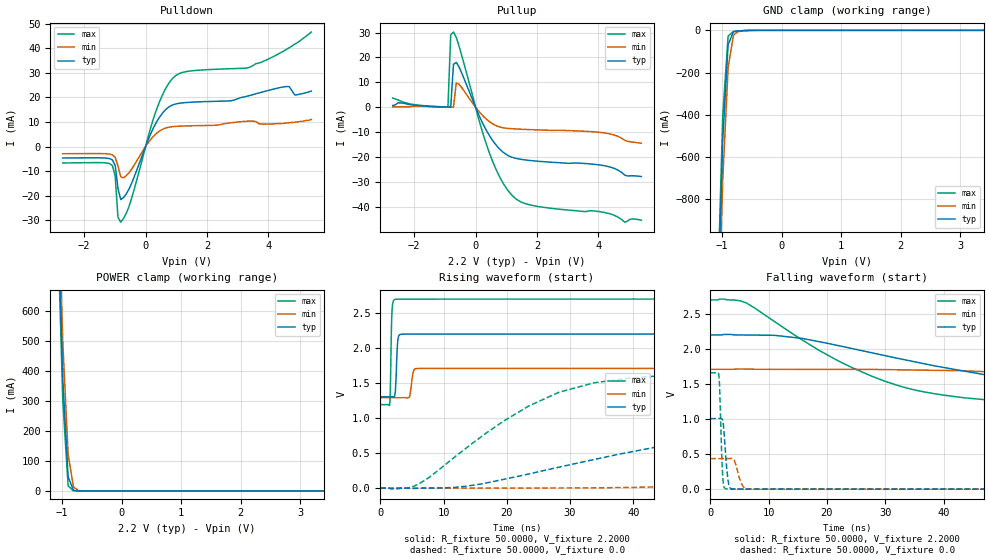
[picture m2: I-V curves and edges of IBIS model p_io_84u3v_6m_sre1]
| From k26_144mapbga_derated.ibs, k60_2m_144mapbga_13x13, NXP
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[Model] p_io_84u3v_6m_sre1
|   Model p_io_84u3v_6m_sre1
| Library cells for typ/min/max conditions are connected as defined below:
|  pad - External Pad
|  ipp_do - Core Input
|  ipp_obe - Output Buffer Enable
|  esd_boost - vdd_s_3v
|  esd_bus - vdd_s_3v
|  ipp_ina40a_3v - NC
|  ipp_ina40b_3v - NC
|  ipp_ina_3v - NC
|  ipp_ind - NC
|  ipp_ind_3v - NC
|  ipp_sre - vdd_s_lv
|  vdd_s_3v - vdd_s_3v
|  vdd_s_lv - vdd_s_lv
|  vss_bulk - vss_bulk
|  vss_s_lv - vss_s_lv
| All other pins connected to ground
Model_type I/O
Polarity   Non-Inverting
Enable   Active-High
Vinl =   0.6600V
Vinh =   1.6500V
Vmeas =  1.1000V
Cref =   25.0000pF
Rref =   50.0000
Vref =   0.0V
C_comp   2.2801pF   2.0930pF   2.5126pF
[Temperature Range]   25.0000   0.1250k   -40.0000
[Voltage Range]   2.2000V   1.7100V   2.7000V
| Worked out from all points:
|   slope of the pulldown table from 0 to 0.33 V, typ, clamps not added: 35.3 ohm
|   slope of the pullup table from 0 to 0.33 V, typ, clamps not added: 37.5 ohm
|   GND clamp passes 1 mA (typ) near -0.60 V on its own axis
|   POWER clamp passes 1 mA (typ) near -0.77 V on its own axis
|   rising waveform, R_fixture 50.0000, V_fixture 2.2000: 20-80 % time 249ps typ, 365ps min, 188ps max; typ from 1.3 V to 2.2 V
|   rising waveform, R_fixture 50.0000, V_fixture 0.0: 20-80 % time 37.7ns typ, 81.3ns min, 17ns max; typ from 0 V to 1.01 V
|   falling waveform, R_fixture 50.0000, V_fixture 2.2000: 20-80 % time 36.7ns typ, 76.7ns min, 20.7ns max; typ from 2.2 V to 1.3 V
|   falling waveform, R_fixture 50.0000, V_fixture 0.0: 20-80 % time 571ps typ, 930ps min, 381ps max; typ from 1.01 V to 0 V
[Pulldown]
|Voltage   I(typ)   I(min)   I(max)
-2.7V     -4.67mA    -2.93mA    -6.69mA
-1.08V    -5.482mA   -3.411mA   -7.784mA
-990mV    -7.73mA    -4.407mA   -11.96mA
-900mV    -17mA      -7.855mA   -28.73mA
-810mV    -21.6mA    -12.32mA   -30.8mA
-540mV    -17.32mA   -10.67mA   -24.41mA
360mV     10.04mA    5.403mA    15.15mA
900mV     17.03mA    8.127mA    28.01mA
3.33V     20.57mA    10.32mA    32.05mA
4.59V     24.4mA     9.6mA      39.55mA
4.86V     21mA       9.9mA      41.7mA
5.4V      22.6mA     11mA       46.6mA
[Pullup]
|Voltage   I(typ)   I(min)   I(max)
-2.7V     700uA      200uA      3.7mA
-900mV    67.5uA     41uA       85.4uA
-810mV    41.47uA    24.4uA     29.06mA
-720mV    17.26mA    23.27uA    30.18mA
-630mV    17.97mA    9.767mA    28.09mA
450mV     -11.38mA   -5.776mA   -18.35mA
810mV     -17.11mA   -8.025mA   -28.58mA
1.17V     -20.02mA   -8.615mA   -35.14mA
1.89V     -21.53mA   -9.048mA   -39.53mA
4.05V     -23.2mA    -10.08mA   -41.95mA
4.86V     -27.27mA   -13.28mA   -46.17mA
5.4V      -27.86mA   -14.46mA   -45.4mA
[GND_clamp]
|Voltage   I(typ)   I(min)   I(max)
-2.7V     -22.06A    -21.95A    -22.16A
-1.08V    -1.367A    -1.534A    -1.279A
-990mV    -516.1mA   -705.4mA   -403.6mA
-900mV    -68.3mA    -177.8mA   -27.24mA
-810mV    -6.453mA   -22.51mA   -5.196mA
-720mV    -2.652mA   -3.714mA   -3.053mA
-450mV    -86.98uA   -164.9uA   -52.14uA
5.4V      0A         0A         0A
[POWER_clamp]
|Voltage   I(typ)   I(min)   I(max)
-2.7V     15.08A     14.99A     15.18A
-1.08V    969.6mA    1.072A     917.9mA
-990mV    374.4mA    496mA      302.2mA
-900mV    47.23mA    122mA      16.99mA
-810mV    1.773mA    12.96mA    214.5uA
-720mV    53.91uA    987.1uA    2.438uA
-630mV    1.624uA    71.95uA    27.87nA
5.4V      0A         0A         0A
[Ramp]
| variable   typ   min   max
dV/dt_r  0.6037/37.7184n   0.2593/81.2449n   0.9957/17.0107n
dV/dt_f  0.5371/36.7111n   0.2505/76.6818n   0.9044/20.7047n
R_load = 50.0000
[Rising Waveform]
R_fixture= 50.0000
V_fixture= 2.2000
V_fixture_min= 1.7100
V_fixture_max= 2.7000
|time   V(typ)   V(min)   V(max)
0s        1.305V     1.291V     1.193V
1.5ns     1.305V     1.291V     1.196V
1.784ns   1.306V     1.291V     2.361V
1.873ns   1.306V     1.291V     2.553V
2.385ns   1.38V      1.291V     2.696V
2.705ns   2.041V     1.291V     2.699V
4.534ns   2.2V       1.293V     2.699V
5.291ns   2.2V       1.683V     2.699V
6.338ns   2.2V       1.709V     2.699V
300ns     2.2V       1.71V      2.7V
[Rising Waveform]
R_fixture= 50.0000
V_fixture= 0.0
V_fixture_min= 0.0
V_fixture_max= 0.0
|time   V(typ)   V(min)   V(max)
0s        1.241nV    38.83nV    72.9pV
6.07ns    -108.7uV   -1mV       58.87mV
19.38ns   123.7mV    46.74uV    951.1mV
28.19ns   298.8mV    1.18mV     1.367V
33.8ns    409.1mV    5.292mV    1.504V
43.85ns   590.3mV    19.17mV    1.602V
70.32ns   886.2mV    107.8mV    1.653V
98.88ns   978mV      218.5mV    1.658V
174.5ns   1.006V     386.4mV    1.659V
300ns     1.006V     432.1mV    1.659V
[Falling Waveform]
R_fixture= 50.0000
V_fixture= 2.2000
V_fixture_min= 1.7100
V_fixture_max= 2.7000
|time   V(typ)   V(min)   V(max)
0s        2.2V       1.71V      2.7V
6.204ns   2.2V       1.714V     2.656V
18.59ns   2.105V     1.71V      1.983V
29.81ns   1.908V     1.706V     1.544V
37.7ns    1.772V     1.697V     1.372V
49.27ns   1.603V     1.67V      1.26V
70.32ns   1.412V     1.597V     1.202V
100.1ns   1.328V     1.482V     1.196V
177.5ns   1.305V     1.325V     1.193V
300ns     1.305V     1.293V     1.193V
[Falling Waveform]
R_fixture= 50.0000
V_fixture= 0.0
V_fixture_min= 0.0
V_fixture_max= 0.0
|time   V(typ)   V(min)   V(max)
0s        1.006V     435.1mV    1.659V
1.462ns   1.006V     434.9mV    1.632V
1.59ns    1.006V     434.8mV    1.482V
1.938ns   1.008V     434.6mV    534.6mV
2.16ns    961.3mV    434.6mV    145.9mV
2.983ns   168mV      435.3mV    1.118mV
3.542ns   6.327mV    438.5mV    292.1uV
5.653ns   68.02uV    34.4mV     309.1uV
7.01ns    93.43uV    931.2uV    257.2uV
300ns     3.061nV    265.4nV    1.191nV
